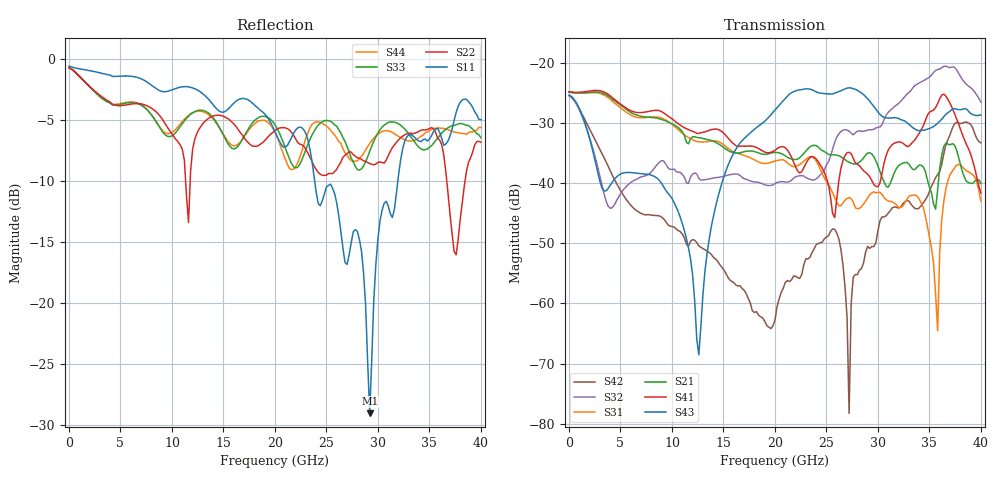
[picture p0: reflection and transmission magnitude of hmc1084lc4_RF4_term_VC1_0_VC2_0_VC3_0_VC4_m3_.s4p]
!Agilent Technologies,N5224A,MY51441122,A.09.40.06
!Agilent N5224A: A.09.40.06
!Date: Thursday, June 19, 2014 00:55:41
!Correction: S11(Full 4 Port(1,2,3,4))
!S12(Full 4 Port(1,2,3,4))
!S13(Full 4 Port(1,2,3,4))
!S14(Full 4 Port(1,2,3,4))
!S21(Full 4 Port(1,2,3,4))
!S22(Full 4 Port(1,2,3,4))
!S23(Full 4 Port(1,2,3,4))
!S24(Full 4 Port(1,2,3,4))
!S31(Full 4 Port(1,2,3,4))
!S32(Full 4 Port(1,2,3,4))
!S33(Full 4 Port(1,2,3,4))
!S34(Full 4 Port(1,2,3,4))
!S41(Full 4 Port(1,2,3,4))
!S42(Full 4 Port(1,2,3,4))
!S43(Full 4 Port(1,2,3,4))
!S44(Full 4 Port(1,2,3,4))
!S4P File: Measurements: <S11,S12,S13,S14>,
!<S21,S22,S23,S24>,
!<S31,S32,S33,S34>,
!<S41,S42,S43,S44>:
# Hz S  dB  R 50
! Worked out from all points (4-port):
!   201 points, 10 MHz to 40 GHz, reference 50 ohm
!   strongest paths, dB at 10 MHz, 10.01 GHz, 20 GHz, 30 GHz, 40 GHz:
!     S43: -25.3, -42.5, -27.8, -28.1, -28.6
!     S41: -24.8, -29.3, -34.5, -40.6, -41.6
!     S21: -24.8, -30.1, -34.9, -37.1, -40.0
!     S31: -24.8, -30.2, -36.3, -41.5, -43.0
!     S32: -25.4, -37.7, -40.1, -30.7, -26.5
!     S42: -25.5, -47.2, -62.7, -47.9, -33.3
!   lowest |S11| = -29.1 dB at 29.2 GHz (marker M1), VSWR 1.07, Z = 47.6 - j2.5 ohm
!   |S11| at or under -10 dB: 23.85 GHz to 31.94 GHz (8.084 GHz wide, 29 % of centre)
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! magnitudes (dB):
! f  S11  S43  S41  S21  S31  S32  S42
! 10 MHz  -0.6  -25.3  -24.8  -24.8  -24.8  -25.4  -25.5
! 12.61 GHz  -2.6  -68.5  -31.7  -32.4  -33.1  -39.2  -50.4
! 15.81 GHz  -3.8  -35.6  -33.2  -34.8  -34.6  -38.5  -56.3
! 25.8 GHz  -11.1  -25.0  -45.7  -35.3  -42.4  -33.2  -47.7
! 27.2 GHz  -16.1  -24.1  -34.8  -36.5  -42.4  -31.3  -78.3
! 29.2 GHz  -29.1  -26.3  -38.9  -34.9  -41.9  -31.1  -50.8
! 40 GHz  -5.0  -28.6  -41.6  -40.0  -43.0  -26.5  -33.3
